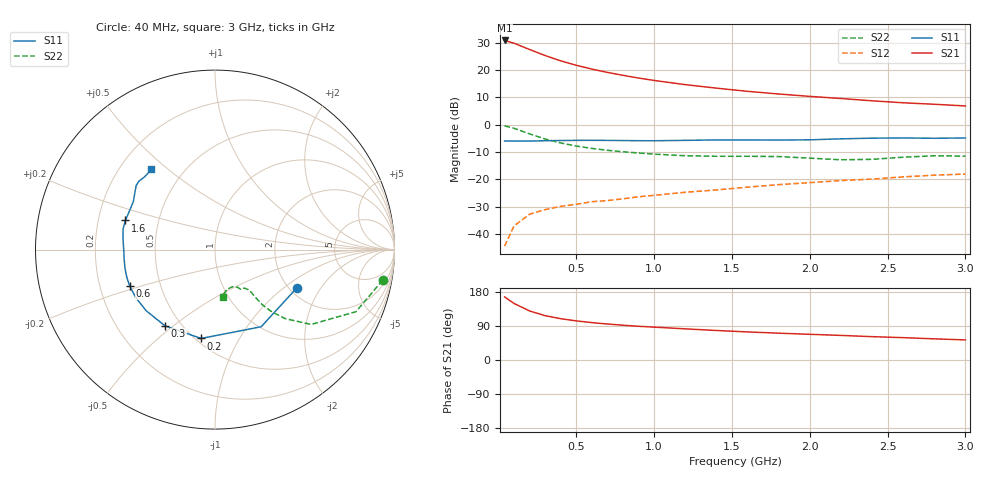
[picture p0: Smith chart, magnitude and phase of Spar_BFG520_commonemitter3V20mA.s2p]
! Filename:  BFG520E.S2P  Version:  2.1
! NXP part #: BFG520  Date: Feb 1992
! Bias condition: Vce=3V, Ic=20mA
! IN LINE PINNING: same data as with cross emitter pinning.
#  MHz  S  MA  R  50
! Freq  S11  S21  S12  S22  !GUM [dB]
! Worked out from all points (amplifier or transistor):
!   21 points, 40 MHz to 3 GHz, reference 50 ohm
!   highest |S21| = 30.8 dB at 40 MHz (marker M1)
!   |S21| within 3 dB of that: start of sweep to 186.9 MHz
!   unconditionally stable (mu >= 1): 889.5 MHz to end of sweep
!   at 300 MHz: K = 0.51, MSG = 28.2 dB, |S12| = -31.1 dB
!   at 1 GHz: K = 1.06, MAG = 19.5 dB, |S12| = -25.8 dB
!   at 3 GHz: K = 1.24, MAG = 9.5 dB, |S12| = -18.1 dB
!   lowest NFmin = 1.45 dB at 500 MHz
!   S11 on the Smith chart (normalised r, x): 40 MHz: 2.18, -1.25; 200 MHz: 0.53, -0.70; 300 MHz: 0.41, -0.47; 600 MHz: 0.33, -0.18; 1.6 GHz: 0.32, +0.14; 3 GHz: 0.33, +0.44
40  0.503 -25.2  34.61 166.5  0.006 78.4  0.95 -10.3
100  0.501 -59.1  30.84 149.3  0.014 68.8  0.858 -23.8
200  0.501 -98.9  23.67 129.5  0.023 57.2  0.679 -37.9
300  0.508 -123.2  18.37 117.0  0.028 53.0  0.547 -44.6
400  0.513 -138.4  14.68 109.0  0.032 52.7  0.463 -47.8
500  0.516 -148.9  12.18 103.2  0.035 52.1  0.406 -49.3
600  0.517 -156.7  10.38 98.7  0.039 53.2  0.368 -49.6
700  0.515 -162.8  9.027 95.0  0.041 54.8  0.34 -49.8
800  0.512 -168.5  7.974 91.8  0.044 56.8  0.319 -49.7
900  0.509 -173.8  7.115 89.0  0.048 59.0  0.303 -49.8
1000  0.508 -178.5  6.434 86.7  0.051 59.8  0.289 -50.4
1200  0.516 173.3  5.39 82.2  0.058 62.2  0.27 -52.6
1400  0.525 167.2  4.652 77.9  0.064 63.3  0.264 -55.5
1600  0.525 162.0  4.064 74.1  0.072 65.7  0.264 -57.0
1800  0.523 155.7  3.634 70.8  0.08 65.8  0.261 -57.4
2000  0.528 149.4  3.289 67.8  0.087 67.1  0.244 -59.1
2200  0.55 144.1  3.006 64.9  0.095 67.2  0.228 -65.1
2400  0.566 140.9  2.729 61.6  0.101 68.4  0.232 -73.7
2600  0.57 138.0  2.511 59.0  0.111 68.4  0.254 -79.0
2800  0.564 134.1  2.359 55.8  0.119 67.2  0.27 -80.0
3000  0.57 128.4  2.196 53.0  0.125 67.9  0.265 -80.8
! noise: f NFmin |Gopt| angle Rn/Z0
500  1.45  0.103  38  0.21
900  1.6  0.104  84  0.22
1000  1.65  0.118  84  0.24
2000  2.2  0.231  -177  0.16
